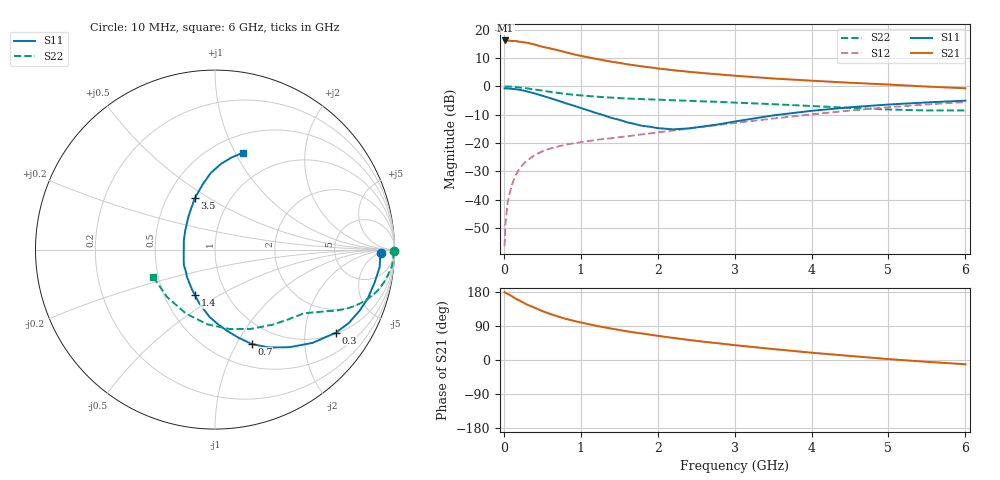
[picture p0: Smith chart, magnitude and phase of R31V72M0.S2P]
! SIEMENS Small Signal Semiconductors
! BFR181
! Si NPN RF Bipolar Junction Transistor in SOT23
! VCE = 1.75 V  IC = 2 mA
! Common Emitter S-Parameters:  May  1996
# GHz  S  MA  R  50
!  f  S11  S21  S12  S22
! GHz  MAG  ANG  MAG  ANG  MAG  ANG  MAG  ANG
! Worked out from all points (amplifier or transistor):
!   36 points, 10 MHz to 6 GHz, reference 50 ohm
!   highest |S21| = 16.3 dB at 20 MHz (marker M1)
!   |S21| within 3 dB of that: start of sweep to 631.5 MHz
!   unconditionally stable (mu >= 1): 1.548 GHz to 3.395 GHz
!   at 250 MHz: K = 0.24, MSG = 21.6 dB, |S12| = -27.6 dB
!   at 1.4 GHz: K = 0.96, MSG = 13.5 dB, |S12| = -18.3 dB
!   at 6 GHz: K = 0.86, MSG = 2.4 dB, |S12| = -5.5 dB
!   S11 on the Smith chart (normalised r, x): 10 MHz: 23, -6; 300 MHz: 1.04, -2.88; 700 MHz: 0.75, -1.16; 1.4 GHz: 0.71, -0.39; 3.5 GHz: 0.69, +0.43; 6 GHz: 0.68, +1.07
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0.01  0.9226 -1.2  6.397 179.0  0.0015 86.5  0.9976 -0.6
0.02  0.9211 -2.4  6.5 177.6  0.0036 90.0  0.994 -1.1
0.05  0.9226 -6.1  6.473 174.4  0.009 87.3  0.9949 -2.8
0.1  0.908 -11.7  6.363 169.0  0.0176 82.4  0.9897 -5.5
0.15  0.894 -17.7  6.376 162.2  0.0262 78.9  0.9744 -8.3
0.3  0.817 -34.5  5.924 146.4  0.0486 70.7  0.9245 -15.2
0.4  0.7521 -43.7  5.497 138.0  0.0608 65.2  0.883 -18.9
0.5  0.6846 -52.6  5.027 129.1  0.0713 61.8  0.8441 -21.7
0.6  0.623 -61.1  4.709 121.7  0.0796 58.5  0.8047 -24.1
0.7  0.5642 -68.8  4.377 115.1  0.0864 56.6  0.7688 -26.0
0.8  0.5068 -75.2  4.034 109.0  0.0929 54.6  0.7392 -27.5
0.9  0.4605 -81.1  3.72 103.7  0.0983 53.8  0.7141 -28.7
1.1  0.3764 -94.6  3.271 94.7  0.1083 52.7  0.6762 -30.9
1.2  0.3396 -100.5  3.073 90.3  0.1132 52.2  0.6606 -32.0
1.4  0.2771 -113.7  2.736 82.7  0.1218 52.4  0.6344 -33.7
1.7  0.2172 -136.1  2.36 72.7  0.1365 53.7  0.603 -36.4
2.2  0.1741 -179.2  1.937 58.3  0.1661 55.0  0.5699 -42.3
2.8  0.2145 136.9  1.63 43.8  0.2093 55.0  0.5339 -51.1
3.5  0.3074 111.5  1.382 28.9  0.2707 52.3  0.4858 -65.4
4.5  0.4281 93.1  1.162 10.7  0.3741 44.0  0.4182 -96.0
5.5  0.5222 79.7  0.995 -4.8  0.4806 31.4  0.3758 -135.3
6  0.5603 74.1  0.928 -11.2  0.5287 24.1  0.3761 -156.3
